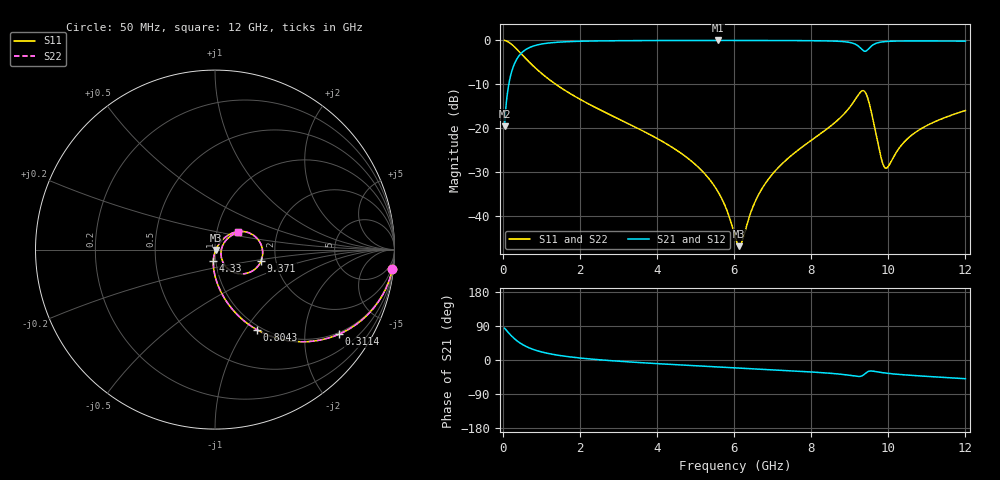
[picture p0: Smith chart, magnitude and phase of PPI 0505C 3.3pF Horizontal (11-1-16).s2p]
# MHz S MA R 50
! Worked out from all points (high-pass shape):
!   1601 points, 50 MHz to 12 GHz, reference 50 ohm
!   highest |S21| = -0.04 dB at 5.577 GHz (marker M1); lowest = -19.6 dB at 50 MHz (marker M2)
!   |S21| within 3 dB of the highest: 471.7 MHz to end of sweep
!   lowest |S11| = -46.9 dB at 6.137 GHz (marker M3), VSWR 1.01, Z = 50.4 - j0.172 ohm
!   |S11| at or under -10 dB: 1.373 GHz to end of sweep
!   |S22| runs from -46.9 to 0.0 dB; largest |S21 - S12| = 0
!   S11 on the Smith chart (normalised r, x): 50 MHz: 1, -19; 311.4 MHz: 0.95, -2.97; 804.3 MHz: 0.95, -1.14; 4.33 GHz: 0.97, -0.12; 9.371 GHz: 1.68, -0.22; 12 GHz: 1.26, +0.25
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50  0.9945 -6.2  0.1044 83.8  0.1044 83.8  0.9945 -6.2
169.5  0.9419 -20.2  0.3354 69.8  0.3354 69.8  0.9419 -20.2
311.4062  0.8362 -34.3  0.5477 55.6  0.5477 55.6  0.8362 -34.3
804.3438  0.5041 -62.4  0.8621 27.5  0.8621 27.5  0.5041 -62.4
1282.344  0.3376 -74.4  0.9392 15.2  0.9392 15.2  0.3376 -74.4
2044.156  0.2082 -84.5  0.9755 4.9  0.9755 4.9  0.2082 -84.5
4038.312  0.07471 -97.2  0.9935 -9.8  0.9935 -9.8  0.07471 -97.2
4329.594  0.0629 -98.2  0.9942 -11.5  0.9942 -11.5  0.0629 -98.2
5076.469  0.03572 -99.3  0.9951 -15.6  0.9951 -15.6  0.03572 -99.3
5576.875  0.01907 -95.6  0.9953 -18.3  0.9953 -18.3  0.01907 -95.6
6025  0.005836 -61.1  0.9952 -20.6  0.9952 -20.6  0.005836 -61.1
6137.031  0.004515 -22.2  0.9951 -21.2  0.9951 -21.2  0.004515 -22.2
6517.938  0.01356 46.0  0.9947 -23.2  0.9947 -23.2  0.01356 46.0
6824.156  0.02383 52.8  0.9942 -24.9  0.9942 -24.9  0.02383 52.8
8019.156  0.07338 52.2  0.9891 -31.7  0.9891 -31.7  0.07338 52.2
9094.656  0.1965 30.2  0.9212 -41.8  0.9212 -41.8  0.1965 30.2
9371  0.2647 -13.4  0.7531 -38.3  0.7531 -38.3  0.2647 -13.4
9512.906  0.1863 -45.9  0.8195 -29.3  0.8195 -29.3  0.1863 -45.9
9849  0.04045 -34.5  0.959 -33.4  0.959 -33.4  0.04045 -34.5
10013.31  0.03732 9.4  0.9726 -35.5  0.9726 -35.5  0.03732 9.4
10685.5  0.08814 41.0  0.9835 -41.1  0.9835 -41.1  0.08814 41.0
12000  0.1583 37.4  0.9777 -49.3  0.9777 -49.3  0.1583 37.4
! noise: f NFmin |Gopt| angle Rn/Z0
50  0.0007011  0.9321  1.726  0.002296
1372  0.005469  0.7521  5.59  0.00444
2701  0.008816  0.7057  9.967  0.00584
4031  0.01184  0.6796  14.37  0.007037
5360  0.01483  0.6651  18.71  0.008273
6682  0.01822  0.6636  22.96  0.009977
8012  0.02475  0.6999  27.2  0.01527
9341  0.1583  0.9384  31.79  0.5306
1.067e+04  0.03538  0.7237  35.81  0.02307
1.2e+04  0.03236  0.675  39.52  0.01709
